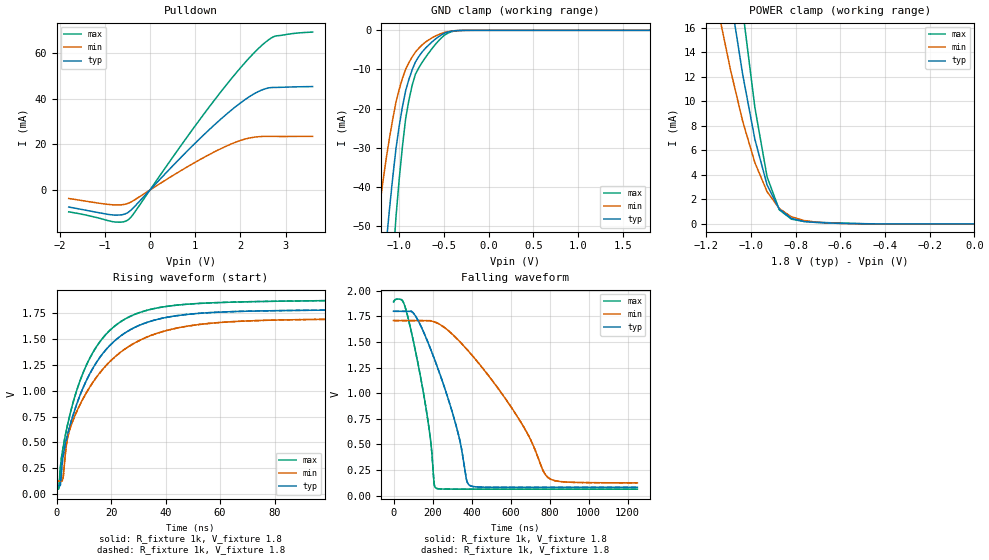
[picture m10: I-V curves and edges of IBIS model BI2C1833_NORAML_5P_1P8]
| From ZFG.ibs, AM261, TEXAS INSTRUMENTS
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[Model]   BI2C1833_NORAML_5P_1P8
Model_type   I/O_open_drain
Polarity   Non-Inverting
Enable   Active-Low
Vinl =  0.54
Vinh =  1.26
Cref =  400pF
Rref =  528
Vref =  1.8V
Vmeas =  0.9
C_comp   2.858406p   2.734081p   3.127023p
|[Input load] normal
|[Output drive] i2c standard
|[supplytol] 5
|[temp] ind
[Model Spec]
Vinl   0.54   0.513   0.567
Vinh   1.26   1.197   1.323
[Temperature Range]   25   125   -40
[Voltage Range]   1.8   1.71   1.89
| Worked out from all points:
|   slope of the pulldown table from 0 to 0.27 V, typ, clamps not added: 47.3 ohm
|   GND clamp passes 1 mA (typ) near -0.51 V on its own axis
|   POWER clamp passes 1 mA (typ) near -0.86 V on its own axis
|   rising waveform, R_fixture 1k, V_fixture 1.8: 20-80 % time 17.4ns typ, 21ns min, 15.1ns max; typ from 0.08 V to 1.8 V
|   rising waveform, R_fixture 1k, V_fixture 1.8: 20-80 % time 17.4ns typ, 21ns min, 15.1ns max; typ from 0.08 V to 1.8 V
|   falling waveform, R_fixture 1k, V_fixture 1.8: 20-80 % time 166ns typ, 334ns min, 96.1ns max; typ from 1.8 V to 0.081 V
|   falling waveform, R_fixture 1k, V_fixture 1.8: 20-80 % time 166ns typ, 334ns min, 96.1ns max; typ from 1.8 V to 0.081 V
| Nom Voltages:
|   VDD=1.1, VDDS=1.8, VDDS18=1.8, ESD_BIASFET=0, VSS=0, VSSS=0
| Min Voltages:
|   VDD=1.045, VDDS=1.71, VDDS18=1.71, ESD_BIASFET=0, VSS=0, VSSS=0
| Max Voltages:
|   VDD=1.16, VDDS=1.89, VDDS18=1.89, ESD_BIASFET=0, VSS=0, VSSS=0
[POWER_clamp]
|   voltage   I(typ)   I(min)   I(max)
-1.8V     125.6mA    90.89mA    174.1mA
-1.127V   23.23mA    15.78mA    33.46mA
-1.073V   16.42mA    11.17mA    23.65mA
-1.055V   14.31mA    9.773mA    20.55mA
-1.036V   12.19mA    8.373mA    17.45mA
-1.018V   10.43mA    7.247mA    14.8mA
-981.8mV  6.903mA    4.997mA    9.497mA
-927.3mV  3.179mA    2.633mA    3.84mA
-872.7mV  1.209mA    1.257mA    1.153mA
-818.2mV  452.5uA    585.6uA    387.6uA
-654.5mV  79.53uA    79.22uA    104.5uA
0V        23.06nA    161nA      231.7nA
[Pulldown]
|   voltage   I(typ)   I(min)   I(max)
-1.8V     -7.503mA   -3.749mA   -9.614mA
-818.2mV  -10.98mA   -6.525mA   -13.94mA
-600mV    -10.81mA   -6.446mA   -14.04mA
-490.9mV  -9.941mA   -5.925mA   -13.2mA
-327.3mV  -6.99mA    -4.193mA   -9.444mA
600mV     12.53mA    7.452mA    17.08mA
1.309V    26.38mA    15.49mA    36.33mA
1.909V    36.72mA    21.03mA    51.36mA
2.345V    42.61mA    23.22mA    60.96mA
2.618V    44.7mA     23.5mA     65.74mA
2.782V    44.96mA    23.46mA    67.52mA
3.6V      45.33mA    23.47mA    69.22mA
[GND_clamp]
|   voltage   I(typ)   I(min)   I(max)
-1.8V     -251.3mA   -159.1mA   -395.2mA
-1.255V   -84.32mA   -51.1mA    -135.4mA
-1.145V   -54.62mA   -32.82mA   -87.84mA
-1.109V   -45.84mA   -27.58mA   -73.48mA
-1.073V   -37.72mA   -22.78mA   -60.15mA
-1.036V   -30.26mA   -18.42mA   -47.83mA
-963.6mV  -19.52mA   -12.26mA   -29.65mA
-927.3mV  -15.37mA   -9.897mA   -22.49mA
-854.5mV  -10.08mA   -6.778mA   -14.01mA
-636.4mV  -3.04mA    -1.976mA   -4.778mA
-345.5mV  -61.12uA   -62.1uA    -91.05uA
1.8V      23.06nA    175.4nA    217.6nA
[Ramp]
| variable   typ   min   max
dV/dt_f  1.0421373/0.1690776u 0.95636594/0.33698972u  1.1137593/98.456538n
dV/dt_r   71.5998m/0.85131504n 65.265563m/1.6966724n 69.079016m/0.59616743n
R_load = 1k
[Rising Waveform]
R_fixture = 1k
V_fixture = 1.8
V_fixture_min = 1.71
V_fixture_max = 1.89
|   time   V(typ)   V(min)   V(max)
0s        80mV       123.9mV    62.24mV
844.7ps   80mV       123.9mV    54.5mV
1.364ns   80mV       123.9mV    243.8mV
2.298ns   344.9mV    141.3mV    432.7mV
3.95ns    562.2mV    526.4mV    658.5mV
6.833ns   825.8mV    764mV      955.1mV
16.43ns   1.343V     1.192V     1.494V
29.89ns   1.629V     1.481V     1.753V
51.66ns   1.75V      1.641V     1.847V
1.25us    1.8V       1.71V      1.89V
[Rising Waveform]
R_fixture = 1k
V_fixture = 1.8
V_fixture_min = 1.71
V_fixture_max = 1.89
|   time   V(typ)   V(min)   V(max)
0s        80mV       123.9mV    62.24mV
844.7ps   80mV       123.9mV    54.5mV
1.364ns   80mV       123.9mV    243.8mV
2.298ns   344.9mV    141.3mV    432.7mV
3.95ns    562.2mV    526.4mV    658.5mV
6.833ns   825.8mV    764mV      955.1mV
16.43ns   1.343V     1.192V     1.494V
29.89ns   1.629V     1.481V     1.753V
51.66ns   1.75V      1.641V     1.847V
1.25us    1.8V       1.71V      1.89V
[Falling Waveform]
R_fixture = 1k
V_fixture = 1.8
V_fixture_min = 1.71
V_fixture_max = 1.89
|   time   V(typ)   V(min)   V(max)
0s        1.8V       1.71V      1.891V
46.45ns   1.8V       1.71V      1.901V
87.78ns   1.8V       1.71V      1.63V
166.6ns   1.542V     1.71V      854.3mV
216.5ns   1.299V     1.692V     74.63mV
319ns     697mV      1.544V     63.42mV
391.3ns   99.06mV    1.396V     63.23mV
640.1ns   80.76mV    755.8mV    63.16mV
795ns     80.69mV    172.6mV    63.16mV
1.25us    80.67mV    124.9mV    63.16mV
[Falling Waveform]
R_fixture = 1k
V_fixture = 1.8
V_fixture_min = 1.71
V_fixture_max = 1.89
|   time   V(typ)   V(min)   V(max)
0s        1.8V       1.71V      1.891V
46.45ns   1.8V       1.71V      1.901V
87.78ns   1.8V       1.71V      1.63V
166.6ns   1.542V     1.71V      854.3mV
216.5ns   1.299V     1.692V     74.63mV
319ns     697mV      1.544V     63.42mV
391.3ns   99.06mV    1.396V     63.23mV
640.1ns   80.76mV    755.8mV    63.16mV
795ns     80.69mV    172.6mV    63.16mV
1.25us    80.67mV    124.9mV    63.16mV
